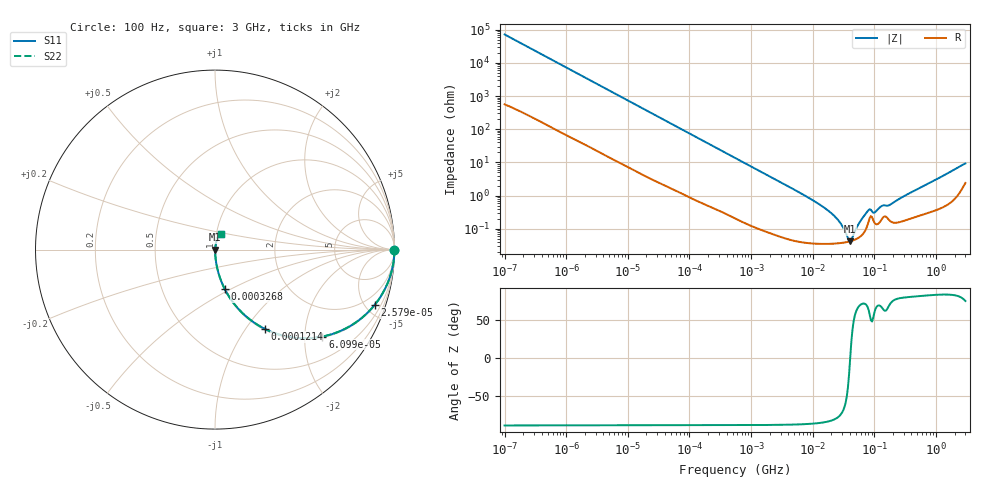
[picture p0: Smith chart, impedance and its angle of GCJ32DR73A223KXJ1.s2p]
!Murata Part Number: GCJ32DR73A223KXJ1
!These Parameters are Measured in Series Mode Connection
!Data Generated on Mar 13, 2026
!  o--ll--o
!Port1  Port2
!  o------o
!Operation Temp=25[degC], DC Bias Voltage=0[V]
!Freq. Start=100[Hz] Stop=3[GHz] 401[Steps]
# Hz S RI R 50
!Freq.(Hz) S11(Real) S11(Imag) S21(Real) S21(Imag) S12(Real) S12(Imag) S22(Real) S22(Imag)
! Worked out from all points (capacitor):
!   401 points, 100 Hz to 3 GHz, reference 50 ohm
!   read as one part in series: C = 22.1 nF near 109 Hz
!   lowest |Z| = 42.2 mohm at 40.54 MHz (marker M1)
!   series resonance near 40.55 MHz, so ESL is about 700 pH
!   S11 on the Smith chart (normalised r, x): 100 Hz: open; 25.79 kHz: 1.06, -5.76; 60.99 kHz: 1.03, -2.45; 121.4 kHz: 1.01, -1.24; 326.8 kHz: 1.01, -0.46; 3 GHz: 1.05, +0.18
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100  1 -0.00139  1.29e-05 0.00139  1.29e-05 0.00139  1 -0.00139
1788  0.9992 -0.0245  0.000831 0.0245  0.000831 0.0245  0.9992 -0.0245
8066  0.9871 -0.1079  0.0129 0.1079  0.0129 0.1079  0.9871 -0.1079
25785  0.8898 -0.308  0.1102 0.308  0.1102 0.308  0.8898 -0.308
31977  0.8412 -0.3603  0.1588 0.3603  0.1588 0.3603  0.8412 -0.3603
60986  0.5987 -0.4845  0.4013 0.4845  0.4013 0.4845  0.5987 -0.4845
121426  0.2787 -0.4424  0.7213 0.4424  0.7213 0.4424  0.2787 -0.4424
326774  0.0537 -0.2183  0.9463 0.2183  0.9463 0.2183  0.0537 -0.2183
547723  0.0208 -0.1356  0.9792 0.1356  0.9792 0.1356  0.0208 -0.1356
1677156  0.00292 -0.0455  0.9971 0.0455  0.9971 0.0455  0.00292 -0.0455
9794414  0.000418 -0.00745  0.9996 0.00745  0.9996 0.00745  0.000418 -0.00745
2.316512e7  0.000365 -0.00227  0.9996 0.00227  0.9996 0.00227  0.000365 -0.00227
2.999103e7  0.000379 -0.00119  0.9996 0.00119  0.9996 0.00119  0.000379 -0.00119
3.71925e7  0.000406 -0.000338  0.9996 0.000338  0.9996 0.000338  0.000406 -0.000338
4.0536e7  0.000422 -1.3e-06  0.9996 1.3e-06  0.9996 1.3e-06  0.000422 -1.3e-06
4.418008e7  0.000443 0.00034  0.9996 -0.00034  0.9996 -0.00034  0.000443 0.00034
5.719833e7  0.000561 0.00144  0.9994 -0.00144  0.9994 -0.00144  0.000561 0.00144
7.730952e7  0.0013 0.00311  0.9987 -0.00311  0.9987 -0.00311  0.0013 0.00311
1.000898e8  0.00155 0.00265  0.9984 -0.00265  0.9984 -0.00265  0.00155 0.00265
1.352818e8  0.0021 0.00453  0.9979 -0.00453  0.9979 -0.00453  0.0021 0.00453
1.751444e8  0.00183 0.00484  0.9982 -0.00484  0.9982 -0.00484  0.00183 0.00484
3e9  0.031 0.0851  0.969 -0.0851  0.969 -0.0851  0.031 0.0851
